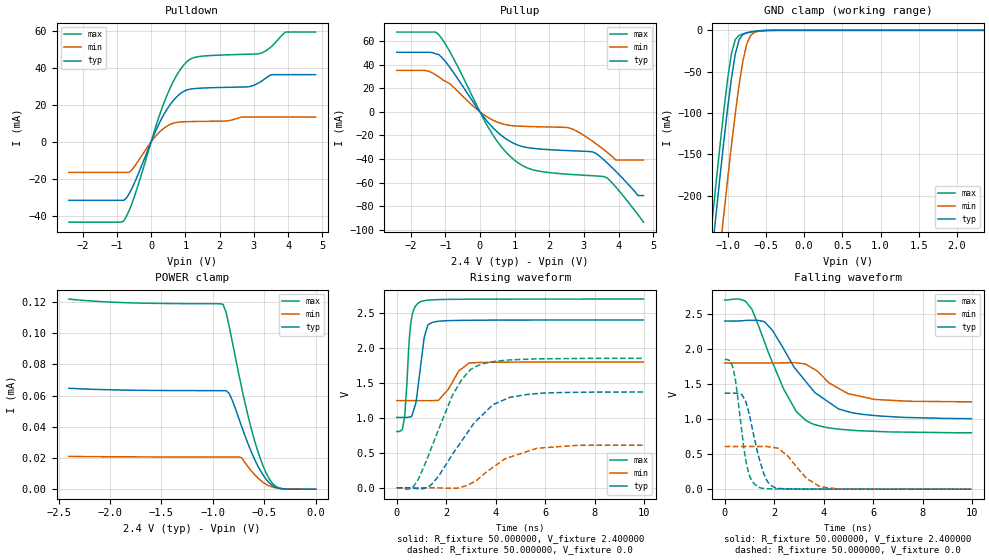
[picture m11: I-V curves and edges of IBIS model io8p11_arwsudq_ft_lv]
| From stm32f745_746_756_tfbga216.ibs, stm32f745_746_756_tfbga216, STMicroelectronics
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|   Model io8p11_arwsudq_ft_lv
[Model]  io8p11_arwsudq_ft_lv
Model_type I/O
Polarity   Non-Inverting
Enable   Active-Low
Vinl =   0.720000V
Vinh =   1.680000V
Vmeas =  1.200000V
Cref =   30.000000pF
Rref =   100.000000M
Vref =   0.0V
C_comp   2.828100pF   2.774600pF   2.917100pF
[Temperature Range]   25.000000   0.125000k   -40.000000
[Pullup Reference]   2.400000V   1.800000V   2.700000V
[Pulldown Reference]   0.0V   0.0V   0.0V
[POWER Clamp Reference]   2.400000V   1.800000V   2.700000V
[GND Clamp Reference]   0.0V   0.0V   0.0V
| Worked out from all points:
|   slope of the pulldown table from 0 to 0.36 V, typ, clamps not added: 25 ohm
|   slope of the pullup table from 0 to 0.36 V, typ, clamps not added: 27.7 ohm
|   GND clamp passes 1 mA (typ) near -0.62 V on its own axis
|   rising waveform, R_fixture 50.000000, V_fixture 2.400000: 20-80 % time 296ps typ, 616ps min, 206ps max; typ from 1.01 V to 2.4 V
|   rising waveform, R_fixture 50.000000, V_fixture 0.0: 20-80 % time 1.73ns typ, 1.71ns min, 1.34ns max; typ from 0 V to 1.37 V
|   falling waveform, R_fixture 50.000000, V_fixture 2.400000: 20-80 % time 1.85ns typ, 1.34ns min, 1.4ns max; typ from 2.4 V to 1.01 V
|   falling waveform, R_fixture 50.000000, V_fixture 0.0: 20-80 % time 557ps typ, 949ps min, 411ps max; typ from 1.37 V to 0 V
[Pulldown]
|Voltage   I(typ)   I(min)   I(max)
-2.4V     -31.67mA   -16.51mA   -43.52mA
-800mV    -31.67mA   -16.51mA   -42.87mA
-480mV    -21.98mA   -13.17mA   -29.21mA
80mV      3.63mA     1.966mA    5.013mA
480mV     18.16mA    8.738mA    26.02mA
800mV     25.38mA    10.72mA    37.77mA
1.12V     28.53mA    11.02mA    44.6mA
2.8V      29.84mA    13.5mA     47.53mA
3.2V      32.66mA    13.5mA     48.04mA
3.52V     36.46mA    13.5mA     51.85mA
3.92V     36.46mA    13.5mA     59.54mA
4.8V      36.46mA    13.5mA     59.54mA
[Pullup]
|Voltage   I(typ)   I(min)   I(max)
-2.4V     50.45mA    35.09mA    67.58mA
-1.52V    50.45mA    34.74mA    67.58mA
-1.2V     48.68mA    29.86mA    65.72mA
320mV     -11.75mA   -6.207mA   -17.08mA
1.04V     -27.54mA   -11.97mA   -41.91mA
1.6V      -31.14mA   -12.58mA   -49.63mA
2.56V     -32.88mA   -13.49mA   -52.9mA
3.28V     -34.2mA    -25.52mA   -54.18mA
3.6V      -41.33mA   -32.62mA   -54.99mA
3.92V     -50.34mA   -40.8mA    -63.66mA
4.56V     -70.9mA    -40.8mA    -87.12mA
4.72V     -70.9mA    -40.8mA    -93.5mA
[GND_clamp]
|Voltage   I(typ)   I(min)   I(max)
-2.4V     -1.425A    -1.508A    -1.394A
-1.25V    -311.8mA   -402mA     -274.5mA
-1.2V     -266mA     -356.2mA   -228.4mA
-1.15V    -220.9mA   -310.9mA   -183.1mA
-1.1V     -176.9mA   -266.3mA   -139mA
-1.05V    -134.3mA   -222.6mA   -97.01mA
-950mV    -57.81mA   -139.1mA   -27.86mA
-900mV    -28.73mA   -100.5mA   -11.04mA
-850mV    -11.29mA   -65.69mA   -6.054mA
-750mV    -2.852mA   -16.6mA    -3.179mA
-600mV    -750uA     -1.167mA   -738.5uA
2.35V     0A         0A         0A
[POWER_clamp]
|Voltage   I(typ)   I(min)   I(max)
-2.4V     64.71uA    21.03uA    121.9uA
-1.86V    63.55uA    20.74uA    119.6uA
-900mV    63.18uA    20.63uA    118.5uA
-870mV    63.14uA    20.63uA    113.2uA
-840mV    61.36uA    20.62uA    104.3uA
-720mV    40.37uA    20.18uA    65.28uA
-630mV    24.69uA    12.08uA    39.85uA
-540mV    12.26uA    5.907uA    20uA
-480mV    6.236uA    3.061uA    10.23uA
-420mV    2.4uA      1.365uA    3.726uA
-360mV    667.9nA    564nA      839.6nA
0V        0A         0A         0A
[Ramp]
| variable   typ   min   max
dV/dt_r  0.82170/1.73045n   0.36406/1.70655n   1.11113/1.33482n
dV/dt_f  0.83244/1.83927n   0.33240/1.35530n   1.13578/1.39484n
R_load = 50.000000
[Rising Waveform]
R_fixture= 50.000000
V_fixture= 2.400000
V_fixture_min= 1.800000
V_fixture_max= 2.700000
|time   V(typ)   V(min)   V(max)
0s        1.006V     1.247V     804.6mV
220.2ps   1.006V     1.247V     829.6mV
300.3ps   1.006V     1.247V     979mV
560.6ps   1.016V     1.247V     2.333V
780.8ps   1.226V     1.247V     2.608V
920.9ps   1.622V     1.247V     2.654V
1.121ns   2.166V     1.247V     2.678V
1.481ns   2.369V     1.247V     2.689V
2.923ns   2.396V     1.785V     2.697V
9.97ns    2.4V       1.8V       2.699V
[Rising Waveform]
R_fixture= 50.000000
V_fixture= 0.0
V_fixture_min= 0.0
V_fixture_max= 0.0
|time   V(typ)   V(min)   V(max)
0s        167.8uV    65.49uV    417.8uV
500.5ps   -1.047mV   52.35uV    -17.76mV
720.7ps   -7.687mV   56.72uV    40.19mV
1.401ns   46.2mV     155.1uV    573.3mV
2.262ns   483.9mV    -7.24mV    1.33V
2.623ns   670.1mV    9.984mV    1.548V
3.183ns   947.3mV    98.67mV    1.733V
3.904ns   1.192V     297.2mV    1.804V
5.666ns   1.347V     566.1mV    1.845V
9.97ns    1.37V      609mV      1.851V
[Falling Waveform]
R_fixture= 50.000000
V_fixture= 2.400000
V_fixture_min= 1.800000
V_fixture_max= 2.700000
|time   V(typ)   V(min)   V(max)
0s        2.4V       1.8V       2.699V
820.8ps   2.407V     1.8V       2.687V
1.101ns   2.41V      1.8V       2.567V
1.602ns   2.392V     1.8V       2.107V
2.382ns   2.002V     1.804V     1.429V
2.903ns   1.698V     1.804V     1.105V
3.283ns   1.534V     1.782V     979.6mV
3.644ns   1.378V     1.706V     921.7mV
5.065ns   1.098V     1.357V     843.2mV
9.97ns    1.006V     1.247V     804.6mV
[Falling Waveform]
R_fixture= 50.000000
V_fixture= 0.0
V_fixture_min= 0.0
V_fixture_max= 0.0
|time   V(typ)   V(min)   V(max)
0s        1.37V      609mV      1.851V
340.3ps   1.37V      609mV      1.728V
440.4ps   1.37V      609mV      1.543V
840.8ps   1.258V     608.9mV    438.5mV
1.041ns   991mV      608.7mV    159.1mV
1.361ns   477.2mV    609mV      30.33mV
1.722ns   113.9mV    607.9mV    6.681mV
2.162ns   12.78mV    581.8mV    3.168mV
3.884ns   1.418mV    32.5mV     1.145mV
9.97ns    167.8uV    65.49uV    417.8uV
